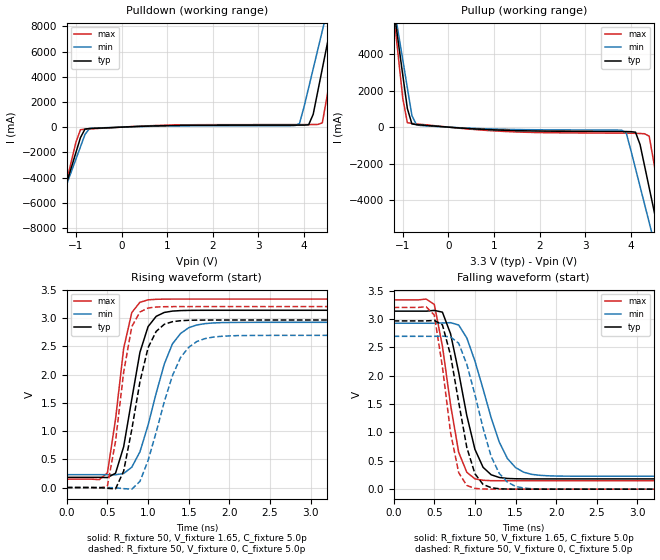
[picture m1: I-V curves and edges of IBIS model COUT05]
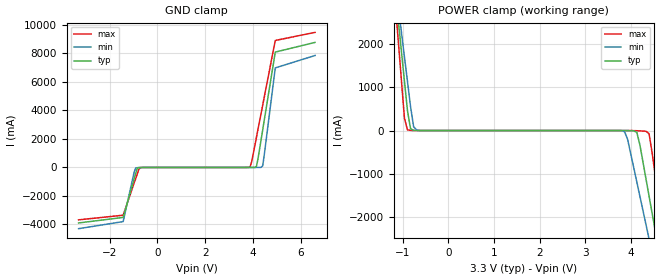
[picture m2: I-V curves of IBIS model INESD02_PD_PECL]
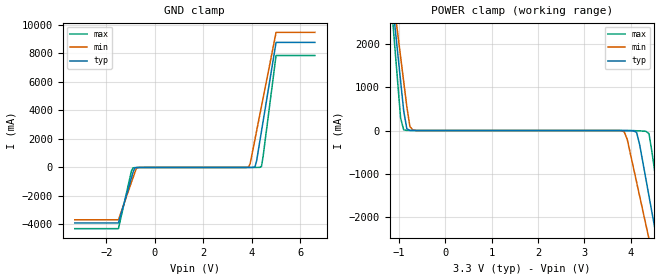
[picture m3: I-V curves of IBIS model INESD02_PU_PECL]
|   This file is an IBIS representation of the   |
|   Integrated Device Technology Inc   |
|   ICS87974i   |
[IBIS Ver]   4.0
[File name]   87974i.ibs
[File Rev]   1.0
[Date]   May  06 2009 | Last Modified
|   May  06 2009 | Generated
[Source] Originated at Integrated Device Technology, Inc.
[Disclaimer]
IDT hereby grants the user of this IBIS model a non-exclusive,
nontransferable license to use this IBIS model under the following terms.
Before using this IBIS model, the user should read this license.
If the user does not accept these terms,  the IBIS model should be
returned to IDT within 30 days.
   The user is granted this license only to use the IBIS model and
is not granted rights to sell, load, rent, lease or license the IBIS
model in whole or in part, or in modified form to anyone other than
user. User may modify the IBIS model to suit its specific
applications but rights to derivative works and such modifications
shall belong to IDT.
   This IBIS model is provided on an "AS IS" basis and IDT makes
absolutely no warranty with respect to the information contained
herein. IDT DISCLAIMS AND CUSTOMER WAIVES ALL WARRANTIES, EXPRESS
OR IMPLIED, INCLUDING WARRANTIES OF MERCHANTABILITY OR FITNESS FOR
A PARTICULAR PURPOSE. The entire risk as to quality and performance
is with the Customer. ACCORDINGLY, IN NO EVENT SHALL THE COMPANY BE
LIABLE FOR ANY DAMAGES, WHETHER IN CONTRACT OR TORT,INCLUDING ANY
LOST PROFITS OR OTHER INCIDENTAL, CONSEQUENTIAL, EXEMPLARY, OR
PUNITIVE DAMAGES ARISING OUT OF THE USE OR APPLICATION OF THE IBIS
model provided in this package. Further, IDT reserves the right to
make changes without notice to any product herein to improve
reliability, function, or design. IDT does not convey any license
under patent rights or any other intellectual property rights,
including those of third parties.
   IDT is not obligated to provide maintenance or support
for the licensed IBIS model.
[Copyright]   Copyright 2009 by Integrated Device Technology, Inc.
[Component]   ICS87974CYI
[Manufacturer] Integrated Device Technology, Inc.
[Package]
|LQFP 52 Pin
|   typ   min   max
R_pkg   52.85m   52.5m   53.2m
L_pkg   3.26nH   2.86nH   3.66nH
C_pkg   0.487pF   0.443pF   0.53pF
[Pin] signal_name   model_name   R_pin   L_pin   C_pin
1   GND   GND   53.20m   3.66n   0.530p
2   nMR/OE   INESD01_PU   53.08m   3.53n   0.523p
3   CLK_EN   INESD01_PU   52.97m   3.39n   0.516p
4   SEL_B   INESD01_PD   52.85m   3.26n   0.509p
5   SEL_C   INESD01_PD   52.73m   3.13n   0.501p
6   PLL_SEL   INESD01_PU   52.62m   2.99n   0.494p
7   SEL_A   INESD01_PD   52.50m   2.86n   0.487p
8   CLK_SEL   INESD01_PD   52.62m   2.99n   0.494p
9   CLK0   INESD02_PD_PECL   52.73m   3.13n   0.501p
10  CLK1   INESD02_PU_PECL   52.85m   3.26n   0.509p
11  nc   nc   52.97m   3.39n   0.516p
12  VDD   POWER   53.08m   3.53n   0.523p
13  VDDA   POWER   53.20m   3.66n   0.530p
14  FB_SEL0   INESD01_PD   53.20m   3.66n   0.530p
15  GND   GND   53.08m   3.53n   0.523p
16  QA4   COUT05   52.97m   3.39n   0.516p
17  VDDOA   POWER   52.85m   3.26n   0.509p
18  QA3   COUT05   52.73m   3.13n   0.501p
19  GND   GND   52.62m   2.99n   0.494p
20  FB_SEL1   INESD01_PD   52.50m   2.86n   0.487p
21  QA2   COUT05   52.62m   2.99n   0.494p
22  VDDOA   POWER   52.73m   3.13n   0.501p
23  QA1   COUT05   52.85m   3.26n   0.509p
24  GND   GND   52.97m   3.39n   0.516p
25  QA0   COUT05   53.08m   3.53n   0.523p
26  VDDOA   POWER   53.20m   3.66n   0.530p
27  nc   nc   53.20m   3.66n   0.530p
28  VDDOFB   POWER   53.08m   3.53n   0.523p
29  QFB   COUT05   52.97m   3.39n   0.516p
30  GND   GND   52.85m   3.26n   0.509p
31  FB_IN   INESD02_PU_PECL   52.73m   3.13n   0.501p
32  QB4   COUT05   52.62m   2.99n   0.494p
33  VDDOB   POWER   52.50m   2.86n   0.487p
34  QB3   COUT05   52.62m   2.99n   0.494p
35  GND   GND   52.73m   3.13n   0.501p
36  QB2   COUT05   52.85m   3.26n   0.509p
37  VDDOB   POWER   52.97m   3.39n   0.516p
38  QB1   COUT05   53.08m   3.53n   0.523p
39  GND   GND   53.20m   3.66n   0.530p
40  QB0   COUT05   53.20m   3.66n   0.530p
41  VDDOB   POWER   53.08m   3.53n   0.523p
42  nc   nc   52.97m   3.39n   0.516p
43  GND   GND   52.85m   3.26n   0.509p
44  QC3   COUT05   52.73m   3.13n   0.501p
45  VDDOC   POWER   52.62m   2.99n   0.494p
46  QC2   COUT05   52.50m   2.86n   0.487p
47  GND   GND   52.62m   2.99n   0.494p
48  QC1   COUT05   52.73m   3.13n   0.501p
49  VDDOC   POWER   52.85m   3.26n   0.509p
50  QC0   COUT05   52.97m   3.39n   0.516p
51  GND   GND   53.08m   3.53n   0.523p
52  VCO_SEL   INESD01_PD   53.20m   3.66n   0.530p
| Models and submodels in the file (5): COUT05 (Output), INESD02_PD_PECL (Input), INESD02_PU_PECL (Input), INESD01_PD (Input), INESD01_PU (Input)
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[Model]   COUT05
Model_type   Output
Polarity   Non-Inverting
|   typ   min   max
C_comp   2pF   1.5pF   2.5pF
Vmeas = 1.65V
Rref = 50
Vref = 1.65V
|   typ   min   max
[Voltage range]   3.3V   3.135V   3.465V
[Pullup Reference]   3.3V   3.135V   3.465V
[Pulldown Reference]   0.0V   0.0V   0.0V
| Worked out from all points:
|   slope of the pulldown table from 0 to 0.495 V, typ, clamps not added: 6.88 ohm
|   slope of the pullup table from 0 to 0.495 V, typ, clamps not added: 5.83 ohm
|   rising waveform, R_fixture 50, V_fixture 1.65, C_fixture 5.0p: 20-80 % time 228ps typ, 327ps min, 182ps max; typ from 0.181 V to 3.14 V
|   falling waveform, R_fixture 50, V_fixture 1.65, C_fixture 5.0p: 20-80 % time 260ps typ, 352ps min, 208ps max; typ from 3.14 V to 0.181 V
|   rising waveform, R_fixture 50, V_fixture 0, C_fixture 5.0p: 20-80 % time 242ps typ, 342ps min, 187ps max; typ from 0 V to 2.97 V
|   falling waveform, R_fixture 50, V_fixture 0, C_fixture 5.0p: 20-80 % time 233ps typ, 304ps min, 195ps max; typ from 2.97 V to 0 V
[pulldown]
|Voltage   I (typ)   I (min)   I (max)
-3.3V     -29.26A    -25.24A    -35.98A
-1.5V     -7.949A    -7.48A     -8.779A
-1.4V     -6.762A    -6.492A    -7.264A
-900mV    -829.9mA   -1.557A    -205.4mA
-700mV    -111.2mA   -105mA     -141mA
3.9V      159.3mA    286.6mA    204.1mA
4.2V      1.015A     4.63A      208mA
4.4V      4.637A     7.645A     337.3mA
4.6V      8.262A     10.66A     4.681A
4.7V      10.08A     12.17A     7A
4.8V      11.89A     13.68A     9.321A
6.6V      44.81A     41.05A     51.4A
[pullup]
|Voltage   I (typ)   I (min)   I (max)
-3.3V     44.73A     38.54A     55.09A
-1.2V     6.49A      6.702A     6.233A
-1.1V     4.667A     5.186A     3.903A
-900mV    1.021A     2.152A     244.4mA
-700mV    135.9mA    120.6mA    176.6mA
3.8V      -238.9mA   -170.1mA   -327.9mA
4.1V      -276.1mA   -2.259A    -337.7mA
4.3V      -2.128A    -4.222A    -361mA
4.4V      -3.308A    -5.204A    -492.7mA
4.6V      -5.67A     -7.17A     -3.414A
4.8V      -8.032A    -9.136A    -6.433A
6.6V      -29.3A     -26.85A    -33.6A
[Ramp]
|   typ   min   max
dV/dt_r   1.98/0.6n   1.98/0.80n   1.98/0.4n
dV/dt_f   1.98/0.6n   1.98/0.80n   1.98/0.4n
[Rising Waveform]
R_fixture = 50
V_fixture = 1.65
V_fixture_max = 1.73
V_fixture_min = 1.57
C_fixture = 5.0p
| Time   typ   min   max
0s        180.7mV    228.1mV    148.5mV
500ps     176.9mV    228.3mV    260.3mV
600ps     254mV      226.3mV    1.212V
700ps     723.5mV    248.7mV    2.467V
800ps     1.567V     361.1mV    3.101V
900ps     2.395V     632.4mV    3.282V
1.1ns     3.033V     1.673V     3.335V
1.3ns     3.126V     2.545V     3.339V
1.6ns     3.14V      2.88V      3.339V
6ns       3.14V      2.927V     3.339V
[Falling Waveform]
R_fixture = 50
V_fixture = 1.65
V_fixture_max = 1.73
V_fixture_min = 1.57
C_fixture = 5.0p
| Time   typ   min   max
0s        3.14V      2.927V     3.339V
500ps     3.154V     2.927V     3.26V
600ps     3.123V     2.932V     2.525V
700ps     2.742V     2.938V     1.49V
800ps     2.06V      2.896V     650.1mV
1ns       702.7mV    2.261V     182.2mV
1.1ns     385.8mV    1.768V     156.6mV
1.3ns     205.9mV    828.8mV    148.9mV
1.6ns     181.7mV    299.2mV    148.5mV
6ns       180.7mV    228.1mV    148.5mV
[Rising Waveform]
R_fixture = 50
V_fixture = 0
V_fixture_max = 0
V_fixture_min = 0
C_fixture = 5.0p
| Time   typ   min   max
0s        694pV      2.926nV    69.28pV
500ps     -13.33mV   493.3uV    29.14mV
600ps     -23.97mV   -4.885mV   818.7mV
700ps     293mV      -19.29mV   2.046V
800ps     1.029V     -28.77mV   2.852V
1ns       2.477V     478.2mV    3.181V
1.2ns     2.893V     1.522V     3.204V
1.4ns     2.956V     2.304V     3.206V
1.7ns     2.967V     2.639V     3.206V
6ns       2.968V     2.696V     3.206V
[Falling Waveform]
R_fixture = 50
V_fixture = 0
V_fixture_max = 0
V_fixture_min = 0
C_fixture = 5.0p
| Time   typ   min   max
0s        2.968V     2.696V     3.206V
500ps     2.977V     2.696V     3.072V
600ps     2.899V     2.7V       2.158V
700ps     2.363V     2.686V     998.4mV
800ps     1.534V     2.575V     291mV
900ps     735.3mV    2.202V     65.39mV
1ns       271.9mV    1.668V     13.56mV
1.2ns     26.21mV    575mV      579.2uV
1.5ns     640.4uV    49.2mV     -8.484uV
6ns       -190.1nV   90.77nV    -131.9nV
[Model]   INESD02_PD_PECL
Model_type  Input
Polarity   Non-Inverting
Vinl = 0.8V
Vinh = 2.0V
|   typ   min   max
C_comp   2pF   1.5pF   2.5pF
|   typ   min   max
[Voltage range]  3.3V   3.15V   3.45V
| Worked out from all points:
|   GND clamp passes 1 mA (typ) near -0.59 V on its own axis
|   POWER clamp passes 1 mA (typ) near -0.70 V on its own axis
[GND_clamp]
-3.3V     -3.894A    -4.294A    -3.674A
-1.434V   -3.506A    -3.799A    -3.352A
-974.8mV  -794.1mA   -331.5mA   -1.096A
-909.1mV  -407.1mA   -35.25mA   -774.3mA
-777.8mV  -10.55mA   -10.84mA   -133.1mA
-646.5mV  -1.912mA   -4.151mA   -2.665mA
3.884V    141.8uA    72.03uA    57.99mA
3.95V     342.2uA    75.94uA    423.8mA
4.146V    78.32mA    440.9uA    2.118A
4.409V    2.651A     112.4mA    4.38A
4.934V    8.093A     6.984A     8.908A
6.6V      8.773A     7.854A     9.475A
[POWER_clamp]
-3.3V     6.7A       6.327A     7.39A
-1.165V   3.23A      3.44A      2.951A
-1.031V   1.843A     2.286A     1.176A
-963.9mV  1.149A     1.709A     289.6mA
-896.9mV  456.5mA    1.133A     15.4mA
-695.9mV  792.2uA    10.73mA    555.6uA
3.861V    -556.7uA   -26.14mA   -39.45uA
4.129V    -41.85mA   -1.19A     -4.904mA
4.33V     -1.119A    -2.176A    -17.86mA
4.531V    -2.305A    -3.163A    -1.019A
4.732V    -3.492A    -4.151A    -2.536A
6.6V      -5.075A    -5.468A    -4.558A
[Model]   INESD02_PU_PECL
Model_type  Input
Polarity   Non-Inverting
Vinl = 0.8V
Vinh = 2.0V
|   typ   min   max
C_comp   2pF   1.5pF   2.5pF
|   typ   min   max
[Voltage range]  3.3V   3.15V   3.45V
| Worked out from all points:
|   GND clamp passes 1 mA (typ) near -0.59 V on its own axis
|   POWER clamp passes 1 mA (typ) near -0.70 V on its own axis
[GND_clamp]
|Voltage   I(typ)   I(min)   I(max)
-3.3V     -3.894A    -3.674A    -4.294A
-1.5V     -3.894A    -3.674A    -4.294A
-963.9mV  -730.3mA   -1.043A    -249.9mA
-896.9mV  -335.4mA   -714.7mA   -27.07mA
-695.9mV  -3.401mA   -10.69mA   -6.477mA
3.861V    50.74uA    27.7mA     7.469uA
3.928V    181.1uA    239mA      10.12uA
4.129V    40.44mA    1.967A     268.6uA
4.196V    445.8mA    2.543A     887.9uA
4.397V    2.525A     4.275A     64.01mA
5V        8.773A     9.475A     7.854A
6.6V      8.773A     9.475A     7.854A
[POWER_clamp]
|Voltage   I(typ)   I(min)   I(max)
-3.3V     6.7A       6.327A     7.39A
-1.165V   3.23A      3.44A      2.951A
-1.031V   1.842A     2.286A     1.176A
-963.9mV  1.149A     1.709A     289.6mA
-896.9mV  456.4mA    1.132A     15.33mA
-695.9mV  727.9uA    10.66mA    491.6uA
3.861V    -620.9uA   -26.2mA    -103.4uA
4.129V    -41.91mA   -1.19A     -4.968mA
4.33V     -1.119A    -2.176A    -17.93mA
4.531V    -2.305A    -3.163A    -1.019A
4.732V    -3.492A    -4.151A    -2.536A
6.6V      -5.075A    -5.469A    -4.558A
